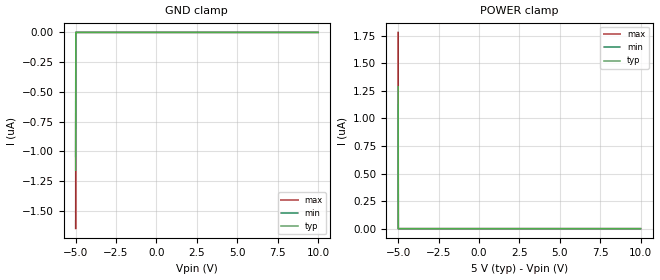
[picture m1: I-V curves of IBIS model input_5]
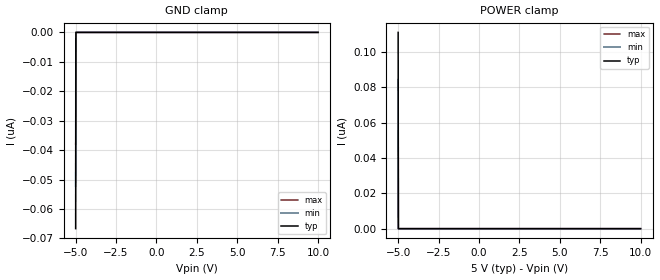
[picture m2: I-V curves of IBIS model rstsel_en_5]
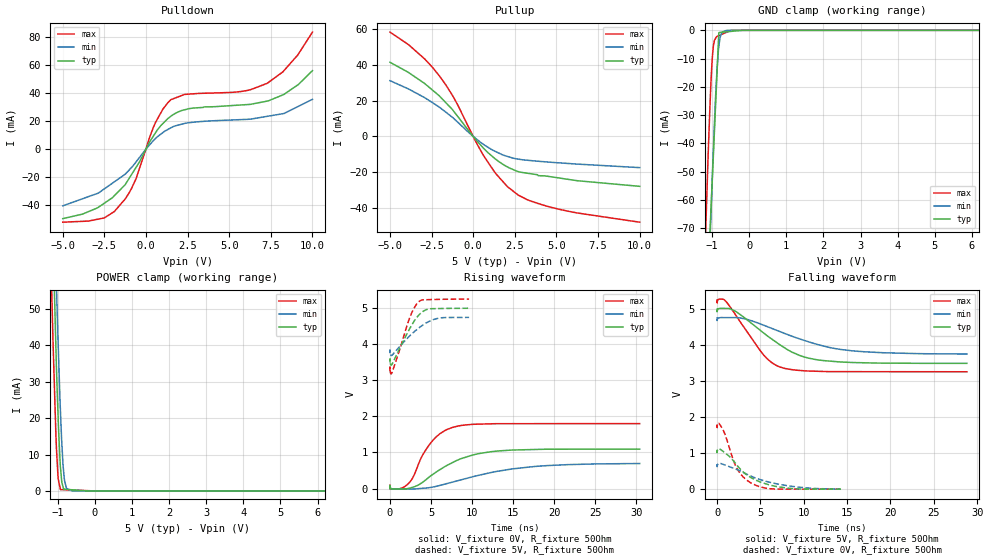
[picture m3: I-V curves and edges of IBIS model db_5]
|Texas Instruments Incorporated
|16-Bit, Single Channel, Parallel Interface with Internal Reference
| Marketing part#   Digital Voltage Range   Package-type   #pins
| DAC7742Y/250   4.75V - 5.25   LQFP   48
| DAC7742Y/250G4   4.75V - 5.25   LQFP   48
| DAC7742YB/250   4.75V - 5.25   LQFP   48
| DAC7742YB/250G4   4.75V - 5.25   LQFP   48
| DAC7742YC/250   4.75V - 5.25   LQFP   48
| DAC7742YC/250G4   4.75V - 5.25   LQFP   48
[IBIS Ver]   3.2
[File name]   dac7742.ibs
|SIMDE Ver   V3.0 - 201101 - RHL4 - Build 424
[File Rev]   1.0
[Date]   10/ 24/ 2011
[Source]
| Texas Instruments Incorporated.
| Analog-eLab Design Center, HPA
| 12500 TI Blvd
| Dallas, TX -75243
| e-mail: elab_scm_ibis@list.ti.com
[Notes]   Revision History:
| Rev 1.0: 10/24/2011
| - Initial version of the model
| - Model generated from simulations in SPECTRE
| - Model matched to SPICE simulation
| - C_comp although listed in numerical order of value are
|   obtained from varying PVT conditions. For PVT conditions for
|   each specific value refer the buffer description under
|   respective [Model]. IBIS model user is responsible for using
|   appropriate C_comp to simulate for Signal Integrity.
| - Model names with a trailing _5 contains the model for
|   5V [4.75V and 5.25V].
[Disclaimer]
| This model is designed as an aid for customers of Texas Instruments.
| TI and its licensors and suppliers make no warranties, either expressed
| or implied, with respect to this  model, including the warranties of
| merchantability or fitness for a particular purpose. The model is
| provided solely on an "as is" basis. The entire risk as to its quality
| and performance is with the customer.
[Copyright]
 (C) Copyright 2011 Texas Instruments Incorporated.All rights reserved.
|   DAC7742PT
[Component]   DAC7742PT
[Manufacturer]   TI
[Package]   |48 LQFP  -  PT package
|   typ   min   max
R_pkg   0.031216   0.01785   0.04507
L_pkg   0.93391nH   0.60773nH   1.24085nH
C_pkg   0.16414pF   0.1401pF   0.20084pF
[Pin]  signal_name   model_name   R_pin   L_pin   C_pin
1   NC   nc   0.02029   0.79829nH  0.17672pF
2   VSS   term_5   0.03716   1.00966nH  0.14794pF
3   VCC   power   0.04055   1.10729nH  0.15413pF
4   VREF   term_5   0.03678   0.99799nH  0.14703pF
5   ROFFSET   term_5   0.03663   0.99344nH  0.14682pF
6   AGND   gnd   0.03714   1.00821nH  0.15065pF
7   AGND   gnd   0.02001   0.79131nH  0.19167pF
8   RFB2   term_5   0.02123   0.85869nH  0.20048pF
9   RFB1   term_5   0.02225   0.91415nH  0.20084pF
10   SJ   term_5   0.04507   1.24085nH  0.16625pF
11   VOUT   term_5   0.02346   1.00389nH  0.19492pF
12   NC   nc   0.03997   1.09593nH  0.13764pF
13   NC   nc   0.04318   1.19076nH  0.14501pF
14   NC   nc   0.04259   1.16808nH  0.15836pF
15   NC   nc   0.03906   1.06267nH  0.14938pF
16   DB0   db_5   0.00056   0.11759nH  0.07856pF
17   DB1   db_5   0.01857   0.66921nH  0.17579pF
18   DB2   db_5   0.00056   0.11755nH  0.07856pF
19   DB3   db_5   0.00056   0.11755nH  0.07856pF
20   DB4   db_5   0.01893   0.67756nH  0.17897pF
21   DB5   db_5   0.00056   0.11760nH  0.07856pF
22   DB6   db_5   0.03752   1.01088nH  0.14479pF
23   NC   nc   0.03944   1.06710nH  0.15121pF
24   NC   nc   0.04235   1.15706nH  0.14307pF
25   NC   nc   0.00056   0.12346nH  0.06703pF
26   TEST   gnd   0.02346   1.00000nH  0.19248pF
27   DB7   db_5   0.04507   1.23285nH  0.16593pF
28   DB8   db_5   0.02225   0.91366nH  0.20049pF
29   DB9   db_5   0.02124   0.85684nH  0.20007pF
30   DB10   db_5   0.02001   0.78838nH  0.19123pF
31   DB11   db_5   0.03714   0.99766nH  0.15023pF
32   DB12   db_5   0.03663   0.98266nH  0.14641pF
33   DB13   db_5   0.03679   0.98729nH  0.14662pF
34   DB14   db_5   0.04055   1.09803nH  0.15379pF
35   DB15   db_5   0.03716   0.99914nH  0.14753pF
36   NC   nc   0.02029   0.78967nH  0.17560pF
37   DGND   gnd   0.04101   1.11801nH  0.14143pF
38   VDD   power   0.03925   1.06168nH  0.14859pF
39   _RST   input_5   0.00056   0.11775nH  0.07855pF
40   _LDAC   input_5   0.01860   0.66582nH  0.18123pF
41   _CS   input_5   0.03513   0.94379nH  0.14577pF
42   R/_W   input_5   0.01785   0.60773nH  0.18642pF
43   RSTSEL   rstsel_en_5   0.03523   0.94652nH  0.14385pF
44   _REFEN   rstsel_en_5   0.03486   0.93889nH  0.14253pF
45   REFOUT   term_5   0.03561   0.96084nH  0.14124pF
46   REFADJ   term_5   0.03491   0.94035nH  0.14010pF
47   REFIN   term_5   0.03619   0.97877nH  0.14445pF
48   NC   nc   0.03891   1.06392nH  0.13839pF
[Model] term_5
Model_type Terminator
C_comp   1.0e-20F  1.0e-20F  1.0e-20F
|   typ   min   max
[Voltage Range]   5V   4.75V   5.25V
[POWER Clamp Reference]   5V   4.75V   5.25V
[GND Clamp Reference]   0V   0V   0V
|Ambient Temperature   25   85   -40
|Junction Temperature
[Temperature Range]   32   92   -40
| Models and submodels in the file (4): input_5 (Input), rstsel_en_5 (Input), db_5 (I/O), term_5 (Terminator)
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|   input_5 Model
[Model]   input_5
Model_type   Input
Vinl = 1.5
Vinh = 3.5
|   typ   min   max
|C_comp from frequency sweep method (F= 25 MHz)
C_comp   1.740e-13   1.707e-13   1.771e-13
|C_comp from LC Tank method (L = 1nH)
|Resonant Frequency(Hz)  1.000e+12   1.000e+12   1.000e+12
|C_comp   2.536e-17   2.536e-17   2.536e-17
| Where nom  PVT is Nominal Process, 5V, 32C
|   Fast PVT is Strong Process,  5.25V, -40C
|   Slow PVT is Weak Process,   4.75V, 92C
[Model Spec]
|Subparameter   typ   min   max
Vinh   3.5   3.325   3.675
Vinl   1.5   1.425   1.575
[Voltage Range]   5   4.75   5.25
|Ambient Temperature   25   85   -40
|Junction Temperature
[Temperature Range]   32   92   -40
[Power Clamp Reference]   5   4.75   5.25
[GND Clamp Reference]   0   0   0
[GND Clamp]
|   Voltage   I(typ)   I(min)   I(max)
-5V       -1.16uA    -1.043uA   -1.65uA
-4.99V    -58.02nA   0A         -157.2nA
-4.99V    0A         0A         -78.58nA
-4.989V   0A         0A         0A
10V       0A         0A         0A
[POWER Clamp]
|   Voltage   I(typ)   I(min)   I(max)
-5V       1.291uA    1.125uA    1.782uA
-4.99V    64.53nA    0A         169.7nA
-4.99V    0A         0A         84.84nA
-4.989V   0A         0A         0A
10V       0A         0A         0A
|   rstsel_en_5 Model
[Model]   rstsel_en_5
Model_type   Input
Vinl = 1.5
Vinh = 3.5
|   typ   min   max
|C_comp from frequency sweep method (F=25MHz)
C_comp   6.430e-14   5.528e-14   6.550e-14
|C_comp from LC tank method (L=1nH)
|Resonant Frequency(Hz)   1.000e+12   1.000e+12   1.000e+12
|C_comp   2.536e-17   2.536e-17   2.536e-17
| Where nom  PVT is Nominal Process, 5V, 32C
|   Fast PVT is Strong Process,  5.25V, -40C
|   Slow PVT is Weak Process,   4.75V, 92C
[Model Spec]
|Subparameter   typ   min   max
Vinh   3.5   3.325   3.675
Vinl   1.5   1.425   1.575
[Voltage Range]   5   4.75   5.25
|Ambient Temperature   25   85   -40
|Junction Temperature
[Temperature Range]   32   92   -40
[Power Clamp Reference]   5   4.75   5.25
[GND Clamp Reference]   0   0   0
[GND Clamp]
|   Voltage   I(typ)   I(min)   I(max)
-5V       -66.7nA    -52.29nA   -37.93nA
-4.995V   -44.47nA   -24.77nA   -37.25nA
-4.995V   -43.35nA   -23.39nA   -37.21nA
-4.99V    -24.46nA   0A         -22.15nA
-4.985V   0A         0A         0A
10V       0A         0A         0A
[POWER Clamp]
|   Voltage   I(typ)   I(min)   I(max)
-5V       111nA      84.37nA    55.33nA
-4.995V   73.68nA    39.96nA    54.7nA
-4.995V   71.84nA    37.74nA    54.67nA
-4.99V    40.53nA    0A         32.54nA
-4.985V   0A         0A         0A
10V       0A         0A         0A
|   db_5 Model
[Model]   db_5
Model_type   I/O
Polarity   Non-Inverting
Enable   Active-High
Vinh = 3.5
Vmeas = 2.5
Vinl = 1.5
Vref = 2.5
Cref = 2pF
Rref = 50
|   typ   min   max
|   (nom PVT)   (fast PVT)   (slow PVT)
|from frequency sweep method (12.5MHz)
C_comp   4.033e-12   3.890e-12   4.146e-12
|Average
|C_comp   4.033e-12   3.890e-12   4.146e-12
|ON state : BUFFER OUTPUT TURNED HIGH
|C_comp (ON state)   5.933e-12   6.162e-12   5.653e-12
|OFF state : BUFFER IN HIGH IMPEDENCE
|C_comp (OFF state)   2.133e-12   2.131e-12   2.126e-12
|C_comp from LC tank measurement(L=1nH)
|C_comp   2.523e-12   2.415e-12   2.622e-12
|ON state : BUFFER OUTPUT TURNED HIGH
|resonant_f(ON)  3.150e+09   3.220e+09   3.090e+09
|C_comp(ON)   2.656e-12   2.555e-12   2.446e-12
|OFF state: BUFFER IN HIGH IMPEDANCE
|resonant_f(OFF) 3.170e+09   3.240e+09   3.110e+09
|C_comp(OFF)   2.523e-12   2.415e-12   2.622e-12
| Where nom  PVT is Nominal Process, 5V, 32C
|   Fast PVT is Strong Process,  5.25V, -40C
|   Slow PVT is Weak Process,   4.75V, 92C
[Model Spec]
|Subparameter   typ   min   max
Vinh   3.5   3.325   3.675
Vinl   1.5   1.425   1.575
[Voltage Range]   5   4.75   5.25
|Ambient Temperature   25   85   -40
|Junction Temperature
[Temperature Range]   32   92   -40
[Pullup Reference]   5   4.75   5.25
[Pulldown Reference]   0   0   0
[Power Clamp Reference]   5   4.75   5.25
[GND Clamp Reference]   0   0   0
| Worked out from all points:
|   slope of the pulldown table from 0 to 0.75 V, typ, clamps not added: 51 ohm
|   slope of the pullup table from 0 to 0.75 V, typ, clamps not added: 96.1 ohm
|   GND clamp passes 1 mA (typ) near -0.82 V on its own axis
|   POWER clamp passes 1 mA (typ) near -0.85 V on its own axis
|   falling waveform, V_fixture 5V, R_fixture 50Ohm: 20-80 % time 5.27ns typ, 7.29ns min, 3.55ns max; typ from 5 V to 3.49 V
|   rising waveform, V_fixture 0V, R_fixture 50Ohm: 20-80 % time 5.07ns typ, 8.37ns min, 2.76ns max; typ from 0 V to 1.09 V
|   rising waveform, V_fixture 5V, R_fixture 50Ohm: 20-80 % time 2.13ns typ, 2.87ns min, 1.72ns max; typ from 3.49 V to 4.99 V
|   falling waveform, V_fixture 0V, R_fixture 50Ohm: 20-80 % time 3.22ns typ, 4.9ns min, 1.9ns max; typ from 1.09 V to 0.002 V
[Pulldown]
|   Voltage   I(typ)   I(min)   I(max)
-5V       -49.78mA   -40.63mA   -52.33mA
-2.91V    -42.05mA   -31.7mA    -50.23mA
-1.903V   -33.39mA   -23.44mA   -44.73mA
-873.5mV  -18.33mA   -13.25mA   -28.34mA
570.3mV   11.65mA    7.538mA    19.03mA
1.505V    23.62mA    15.29mA    35.43mA
2.8V      29.34mA    19.17mA    39.53mA
5.804V    31.65mA    21.15mA    41.39mA
7.28V     34.34mA    23.44mA    47.07mA
8.22V     38.79mA    25.33mA    55.25mA
9.117V    45.93mA    30.37mA    67.35mA
10V       56.16mA    35.62mA    83.75mA
[GND Clamp]
|   Voltage   I(typ)   I(min)   I(max)
-5V       -1.86A     -1.866A    -1.85A
-1.246V   -127.5mA   -151.3mA   -101.1mA
-1.11V    -86.99mA   -96.31mA   -45.42mA
-1.048V   -68.66mA   -71.55mA   -23.79mA
-1.036V   -65.17mA   -67.27mA   -20.06mA
-962.7mV  -43.34mA   -41.28mA   -5.27mA
-867.5mV  -15.06mA   -13.87mA   -2.174mA
-820mV    -953.5uA   -5.861mA   -1.897mA
-810mV    -772.6uA   -4.881mA   -1.839mA
-734.5mV  -679.3uA   -625.8uA   -1.399mA
-611mV    -526.6uA   -14.37uA   -680uA
10V       0A         0A         0A
[Pullup]
|   Voltage   I(typ)   I(min)   I(max)
-5V       41.34mA    31.08mA    58.14mA
-3.887V   35.63mA    26.43mA    51.16mA
-2.9V     29.36mA    21.5mA     43.04mA
-2.029V   22.52mA    16.28mA    33.7mA
-1.036V   12.4mA     8.85mA     19.39mA
649mV     -6.87mA    -4.67mA    -11.08mA
1.353V    -12.74mA   -8.455mA   -20.7mA
2.056V    -17.02mA   -11.17mA   -28.01mA
2.717V    -19.64mA   -12.68mA   -32.79mA
3.868V    -21.38mA   -13.82mA   -37.31mA
5.374V    -23.48mA   -14.88mA   -41.05mA
10V       -27.84mA   -17.41mA   -47.82mA
[POWER Clamp]
|   Voltage   I(typ)   I(min)   I(max)
-5V       1.808A     1.821A     1.801A
-1.246V   115.1mA    138.9mA    88.41mA
-1.125V   68.88mA    91.33mA    40.82mA
-1.067V   46.5mA     68.27mA    21.55mA
-1.025V   31mA       53.29mA    10.06mA
-989mV    20.38mA    40.96mA    3.432mA
-926mV    6.529mA    21.94mA    368.4uA
-858mV    1.185mA    7.434mA    341.3uA
-815.3mV  466.8uA    2.846mA    324.2uA
-763mV    428.1uA    697uA      303.4uA
-611mV    315.5uA    4.12uA     242.8uA
10V       0A         0A         0A
[Ramp]
R_load = 50
|   typ   min   max
dV/dt_r   0.65707/5.03128e-09   0.418482/8.40529e-09   1.07968/2.76479e-09
dV/dt_f   0.905576/5.27111e-09   0.602004/7.29983e-09   1.19651/3.55394e-09
[Falling Waveform]
V_fixture = 5V
V_fixture_min = 4.75V
V_fixture_max = 5.25V
R_fixture = 50Ohm
|   Time   V(typ)   V(min)   V(max)
0s        5V         4.75V      5.25V
1ps       4.922V     4.678V     5.166V
805.4ps   5.016V     4.762V     5.256V
1.989ns   4.953V     4.76V      4.885V
5.244ns   4.357V     4.561V     3.759V
7.262ns   4.003V     4.371V     3.389V
9.516ns   3.711V     4.17V      3.295V
12.31ns   3.568V     3.97V      3.266V
17.03ns   3.507V     3.813V     3.261V
28.82ns   3.492V     3.75V      3.258V
[Rising Waveform]
V_fixture = 0V
V_fixture_min = 0V
V_fixture_max = 0V
R_fixture = 50Ohm
|   Time   V(typ)   V(min)   V(max)
0s        113.1pV    139pV      85.61pV
1ps       88.78mV    78.67mV    100.5mV
110.7ps   444.8uV    4.288mV    -7.627mV
900.1ps   -13.85mV   -11.36mV   -17.37mV
2.189ns   202.8uV    -11.99mV   124.5mV
4.981ns   354.7mV    31.86mV    1.268V
7.517ns   706.9mV    172.4mV    1.686V
13.33ns   1.044V     486.2mV    1.796V
19.22ns   1.089V     636.5mV    1.797V
30.42ns   1.092V     693.1mV    1.798V
[Rising Waveform]
V_fixture = 5V
V_fixture_min = 4.75V
V_fixture_max = 5.25V
R_fixture = 50Ohm
|   Time   V(typ)   V(min)   V(max)
0s        3.491V     3.746V     3.256V
1ps       3.593V     3.84V      3.369V
30.99ps   3.489V     3.753V     3.252V
97.23ps   3.425V     3.696V     3.183V
236.4ps   3.438V     3.691V     3.208V
2.344ns   4.402V     4.215V     4.695V
3.479ns   4.796V     4.441V     5.17V
4.613ns   4.969V     4.613V     5.232V
5.84ns    4.985V     4.715V     5.24V
9.64ns    4.994V     4.741V     5.249V
[Falling Waveform]
V_fixture = 0V
V_fixture_min = 0V
V_fixture_max = 0V
R_fixture = 50Ohm
|   Time   V(typ)   V(min)   V(max)
0s        1.095V     698mV      1.799V
1ps       1.015V     626.2mV    1.709V
186.4ps   1.12V      713.6mV    1.829V
805.4ps   1.026V     679.6mV    1.582V
1.817ns   805.3mV    588.1mV    841.3mV
2.344ns   648.9mV    540.3mV    551mV
4.084ns   298.4mV    344.8mV    148.7mV
5.807ns   135.1mV    208.4mV    21.98mV
8.149ns   28.97mV    96.66mV    1.643mV
14.28ns   2.176mV    2.765mV    1.327mV
